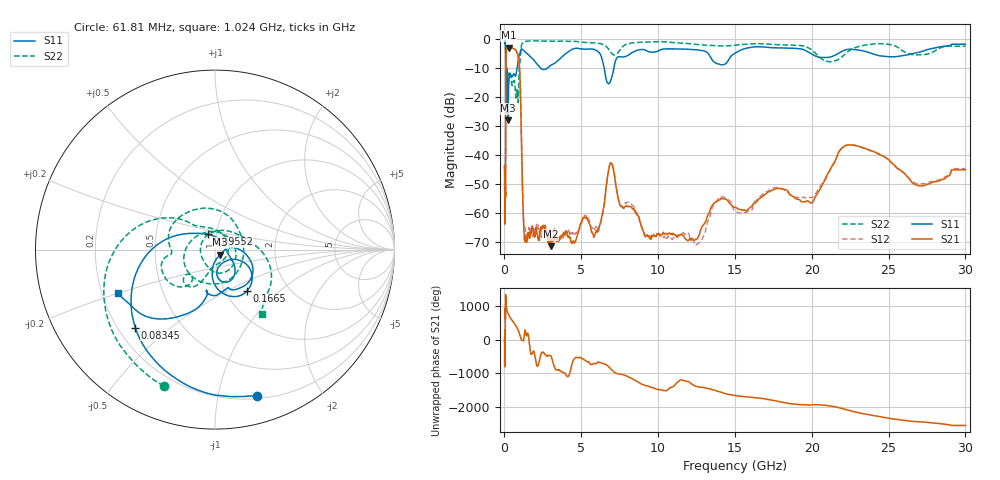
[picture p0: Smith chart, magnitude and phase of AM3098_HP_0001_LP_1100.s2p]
! Date/Time: Thu, Feb 28, 2019 8:32 AM
! Network Analyzer: Agilent Technologies E8364B Rev: A.07.50.67
! Sweep from 0.010 to 30.000 GHz, 1601 Points, Sweep Type: LOG
! Power Supply: 5.023 V, 0.002 A
# Hz S DB R 50
!freq MagS11 AngS11 MagS21 AngS21 MagS12 AngS12 MagS22 AngS22
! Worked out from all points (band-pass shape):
!   1601 points, 10 MHz to 30 GHz, reference 50 ohm
!   highest |S21| = -2.78 dB at 267.8 MHz (marker M1); lowest = -71.3 dB at 3.002 GHz (marker M2)
!   |S21| within 3 dB of the highest: 105.6 MHz to 887.5 MHz (781.9 MHz wide, 157 % of centre)
!   lowest |S11| = -27.9 dB at 232.8 MHz (marker M3), VSWR 1.08, Z = 53 - j2.92 ohm
!   |S11| at or under -10 dB: 91.06 MHz to 811.5 MHz (720.4 MHz wide, 160 % of centre); 2.374 GHz to 2.772 GHz (397.8 MHz wide, 15.5 % of centre); 6.497 GHz to 7.119 GHz (622 MHz wide, 9.14 % of centre)
!   |S22| runs from -22.8 to -0.5 dB; largest |S21 - S12| = 0.012
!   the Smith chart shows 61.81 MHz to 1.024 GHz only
!   S11 on the Smith chart (normalised r, x): 61.81 MHz: 0.23, -1.31; 83.45 MHz: 0.27, -0.38; 95.52 MHz: 0.91, +0.16; 166.5 MHz: 1.25, -0.63; 1.024 GHz: 0.26, -0.20
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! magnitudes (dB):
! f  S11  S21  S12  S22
! 10 MHz  -0.3  -44.4  -43.9  -0.6
! 38.04 MHz  -0.5  -60.8  -59.4  -1.0
! 61.81 MHz  -1.4  -53.1  -53.5  -1.8
! 83.45 MHz  -4.1  -31.3  -31.2  -4.6
! 95.52 MHz  -20.5  -10.2  -10.2  -22.1
! 144.7 MHz  -14.7  -3.4  -3.4  -12.7
! 166.5 MHz  -10.7  -3.3  -3.3  -10.1
! 232.8 MHz  -27.9  -2.9  -2.8  -12.1
! 267.8 MHz  -16.9  -2.8  -2.8  -12.3
! 550.5 MHz  -12.3  -3.1  -3.0  -14.9
! 885.5 MHz  -7.8  -5.7  -5.7  -21.7
! 1.024 GHz  -4.5  -14.8  -14.7  -7.0
! 1.295 GHz  -4.1  -68.5  -64.6  -0.8
! 2.084 GHz  -8.2  -65.2  -63.8  -0.5
! 3.002 GHz  -9.0  -71.3  -67.5  -0.6
! 5.959 GHz  -3.7  -66.4  -64.5  -1.2
! 6.924 GHz  -14.0  -42.6  -42.5  -4.4
! 7.926 GHz  -5.8  -57.3  -56.4  -1.7
! 12.56 GHz  -3.6  -68.8  -70.5  -1.8
! 19.8 GHz  -4.4  -55.9  -54.5  -3.0
! 22.56 GHz  -3.4  -36.4  -36.4  -3.5
! 30 GHz  -1.7  -45.0  -44.6  -2.3
